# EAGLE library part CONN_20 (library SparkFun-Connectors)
Multi connection point. Often used as Generic Header-pin footprint for 0.1 inch spaced/style header connections On any of the 0.1 inch spaced packages, you can populate with these: Break Away Headers - Straight (PRT-00116) Break Away Male Headers - Right Angle (PRT-00553) Female Headers (PRT-00115) Break Away Headers - Machine Pin (PRT-00117) Break Away Female Headers - Swiss Machine Pin (PRT-00743) For SCREWTERMINALS and SPRING TERMINALS visit here: Screw Terimnals on SparkFun.com (5mm/3.5mm/2.54mm spacing) This device is also useful as a general connection point to wire up your design to another part of your project. Our various solder wires solder well into these plated through hole pads. Hook-Up Wire - Assortment (Stranded, 22 AWG) (PRT-11375) Hook-Up Wire - Assortment (Solid Core, 22 AWG) (PRT-11367) View the entire wire category on our website here Special notes: Molex polarized connector foot print use with SKU : PRT-08231 with associated crimp pins and housings. 1MM SMD Version SKU: PRT-10208 NOTES ON THE VARIANTS LOCK and LOCK_LONGPADS... This footprint was designed to help hold the alignment of a through-hole component (i.e. 6-pin header) while soldering it into place. You may notice that each hole has been shifted either up or down by 0.005 of an inch from it's more standard position (which is a perfectly straight line). This slight alteration caused the pins (the squares in the middle) to touch the edges of the holes. Because they are alternating, it causes a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
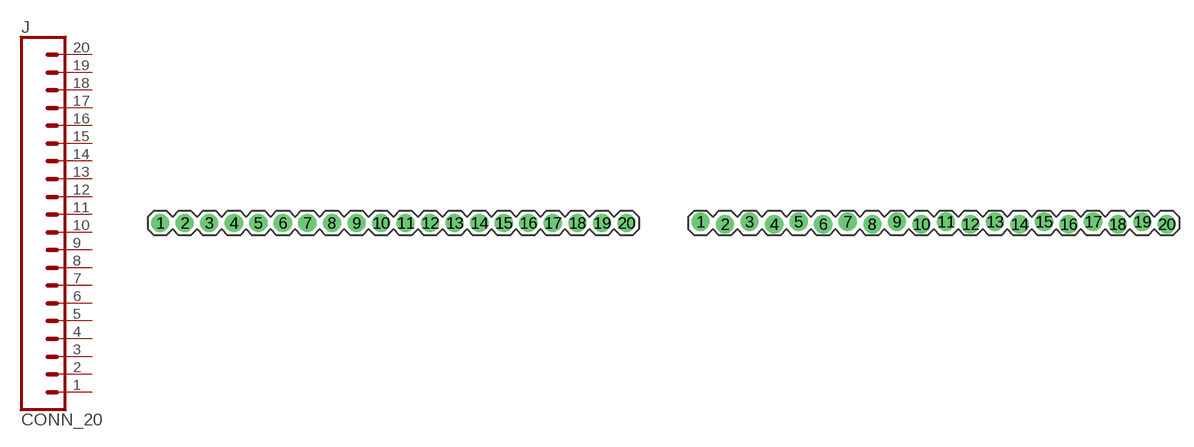
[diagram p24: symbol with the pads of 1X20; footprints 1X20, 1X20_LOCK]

Designator prefix J

## CONN_20  [1X20]
1  1  pas
2  2  pas
3  3  pas
4  4  pas
5  5  pas
6  6  pas
7  7  pas
8  8  pas
9  9  pas
10  10  pas
11  11  pas
12  12  pas
13  13  pas
14  14  pas
15  15  pas
16  16  pas
17  17  pas
18  18  pas
19  19  pas
20  20  pas

## CONN_20LOCK  [1X20_LOCK]
Pads as for 1X20

## CONN_20LOCK_LONGPADS  [1X20_LOCK_LONGPADS]
Pads as for 1X20

## CONN_20SPECIAL  [1X20_LOCK_SPECIAL]
Pads as for 1X20

## CONN_20NO_SILK_KIT  [1X20_NO_SILK_KIT]
Pads as for 1X20

## CONN_20LOCK_NOSILK (PROD_ID: CONN-09864)  [1X20_LOCK_NOSILK]
Pads as for 1X20

## CONN_20NOSILK  [1X20_NOSILK]
Pads as for 1X20

## Footprint 1X20 (pad centres in mm)
Plated Through Hole -20 Pin Specifications: Pin count:20 Pin pitch:0.1" Example device(s): CONN_20
drill 1.016 pad 1.88: 1 0,0; 2 2.54,0; 3 5.08,0; 4 7.62,0; 5 10.16,0; 6 12.7,0; 7 15.24,0; 8 17.78,0; 9 20.32,0; 10 22.86,0; 11 25.4,0; 12 27.94,0; 13 30.48,0; 14 33.02,0; 15 35.56,0; 16 38.1,0; 17 40.64,0; 18 43.18,0; 19 45.72,0; 20 48.26,0

## Footprint 1X20_LOCK (pad centres in mm)
Plated Through Hole -20 Pin Locking Footprint Holes are offset 0.005" from center to hold pins in place while soldering. Specifications: Pin count:20 Pin pitch:0.1" Example device(s): CONN_20
drill 1.016 pad 1.88: 1 0,0.127; 2 2.54,-0.127; 3 5.08,0.127; 4 7.62,-0.127; 5 10.16,0.127; 6 12.7,-0.127; 7 15.24,0.127; 8 17.78,-0.127; 9 20.32,0.127; 10 22.86,-0.127; 11 25.4,0.127; 12 27.94,-0.127; 13 30.48,0.127; 14 33.02,-0.127; 15 35.56,0.127; 16 38.1,-0.127; 17 40.64,0.127; 18 43.18,-0.127; 19 45.72,0.127; 20 48.26,-0.127

## Footprint 1X20_LOCK_LONGPADS (pad centres in mm)
Plated Through Hole -20 Pin Locking Footprint Long Pads Holes are offset 0.005" from center to hold pins in place while soldering. Specifications: Pin count:20 Pin pitch:0.1" Example device(s):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
drill 1.016 long: 1 0,0.127; 2 2.54,-0.127; 3 5.08,0.127; 4 7.62,-0.127; 5 10.16,0.127; 6 12.7,-0.127; 7 15.24,0.127; 8 17.78,-0.127; 9 20.32,0.127; 10 22.86,-0.127; 11 25.4,0.127; 12 27.94,-0.127; 13 30.48,0.127; 14 33.02,-0.127; 15 35.56,0.127; 16 38.1,-0.127; 17 40.64,0.127; 18 43.18,-0.127; 19 45.72,0.127; 20 48.26,-0.127

## Footprint 1X20_LOCK_SPECIAL (pad centres in mm)
Plated Through Hole -20 Pin Locking Footprint Holes are offset 0.005" from center to hold pins in place while soldering. Specifications: Pin count:20 Pin pitch:0.1" Example device(s): CONN_20
drill 1.016 pad 1.88: 1 0,0.127; 2 2.54,-0.127; 3 5.08,0.127; 4 7.62,-0.127; 5 10.16,0.127; 6 12.7,-0.127; 7 15.24,0.127; 8 17.78,-0.127; 9 20.32,0.127; 10 22.86,-0.127; 11 25.4,0.127; 12 27.94,-0.127; 13 30.48,0.127; 14 33.02,-0.127; 15 35.56,0.127; 16 38.1,-0.127; 17 40.64,0.127; 18 43.18,-0.127; 19 45.593,0; 20 48.387,0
